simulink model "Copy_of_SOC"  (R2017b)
settings: Solver=FixedStepDiscrete  StartTime=0.0  StopTime=10.0  FixedStep=0.01  RelTol=1e-3  EnableMultiTasking=on
undefined symbols (not defined in the file): ASWTYPE_FALSE, ASWTYPE_TRUE, CaSOC_OneSOCVoltTable_mV, CaSOC_ZeroSOCTempTable_C, CaSOC_ZeroSOCVoltTable_mV, CbSOC_ManualDeplaCorrect_flg, CbSOC_ManuOCVCorrect_flg, CbSOC_SOCHighDiagOn_flg, CbSOC_SOCLowDiagOn_flg, CcSOC_ACChrgFinishDispSOC_pct, CcSOC_ACChrgFinishMaxSOC_pct, CcSOC_ACStepChrgMaxSOC_pct, CcSOC_AllowMaxCellSOC_pct, CcSOC_AllowMinCellSOC_pct, CcSOC_CapCalcCycl_ms, CcSOC_CellMinTempFilterAvg_numb, CcSOC_CellVoltMeasTol_mV, CcSOC_ChrgFishBefMaxSOC_pct, CcSOC_ChrgFishBefMinSOC_pct, CcSOC_ChrgFollowCurr_A, CcSOC_DCChrgFinishDispSOC_pct, CcSOC_DCChrgFinishMaxSOC_pct, CcSOC_DCStepChrgMaxSOC_pct, CcSOC_DeplaCellVoltMeasTol_mV, CcSOC_DeplaCorrectSOCDiff_pct, CcSOC_DisChrgFlwCurr_A, CcSOC_DispSOCChgSleepTime_min, CcSOC_DispSOCCordRunTi_ms, CcSOC_DispSOCErr_pct, CcSOC_FlwTarSOCDiff_pct, CcSOC_FullChrgTempThrld_C, CcSOC_MaxFlwDispSOC_pct, CcSOC_MinFlwDispSOC_pct, CcSOC_OCVCorrectRunTime_ms, CcSOC_OCVCorrectSleepTime_min, CcSOC_OCVCorrectSOCDiff_pct, CcSOC_OCVPeakCellVoltDev_mV, CcSOC_OCVPeakCellVoltTime_ms, CcSOC_PackSOCUseMax_pct, CcSOC_PackSOCUseMin_pct, CcSOC_SOCDeplaCurrThrd_A, CcSOC_SOCDeplaCurrThrdTi_ms, CcSOC_SOCDeplaNoOCVTi_min, CcSOC_SOCDeplaOCVTi_min, CcSOC_SOCHighAlarmThrld_pct, CcSOC_SOCHighWarningThrld_pct, CcSOC_SOCHysValue_pct, CcSOC_SOCLowAlarmThrld_pct, CcSOC_SOCLowWarningThrld_pct, CcSOC_ZeroMinSOC_pct, CcSOC_ZeroPackCrntThrd_A, CcSOC_ZeroSOCRunTime_ms, Enum_CTCCtrCtlConnMode, Enum_MSMBMUState, SOC_CONST0_NUMB, SOC_CONST1000_NUMB, SOC_CONST100_NUMB, SOC_CONST2080_NUMB, SOC_CONST3600000_NUMB, SOC_CONST60000_NUMB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
libraries: AIWAYS_Powertrain_BMS_lib x109
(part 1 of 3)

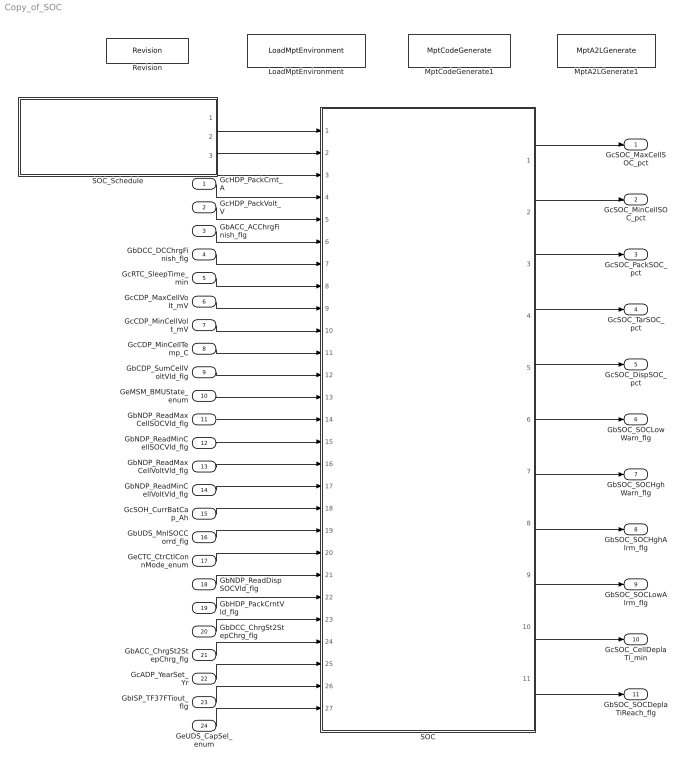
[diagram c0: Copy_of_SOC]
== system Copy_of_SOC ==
  GcHDP_PackCrnt_A : Inport
  GcHDP_PackVolt_V : Inport  Port=2
  GbACC_ACChrgFinish_flg : Inport  Port=3
  GbDCC_DCChrgFinish_flg : Inport  Port=4
  GcRTC_SleepTime_min : Inport  Port=5
  GcCDP_MaxCellVolt_mV : Inport  Port=6
  GcCDP_MinCellVolt_mV : Inport  Port=7
  GcCDP_MinCellTemp_C : Inport  Port=8
  GbCDP_SumCellVoltVld_flg : Inport  Port=9
  GeMSM_BMUState_enum : Inport  Port=10
  GbNDP_ReadMaxCellSOCVld_flg : Inport  Port=11
  GbNDP_ReadMinCellSOCVld_flg : Inport  Port=12
  GbNDP_ReadMaxCellVoltVld_flg : Inport  Port=13
  GbNDP_ReadMinCellVoltVld_flg : Inport  Port=14
  GcSOH_CurrBatCap_Ah : Inport  Port=15
  GbUDS_MnlSOCCorrd_flg : Inport  Port=16
  GeCTC_CtrCtlConnMode_enum : Inport  Port=17
  GbNDP_ReadDispSOCVld_flg : Inport  Port=18
  GbHDP_PackCrntVld_flg : Inport  Port=19
  GbDCC_ChrgSt2StepChrg_flg : Inport  Port=20
  GbACC_ChrgSt2StepChrg_flg : Inport  Port=21
  GcADP_YearSet_Yr : Inport  Port=22
  GbISP_TF37FTiout_flg : Inport  Port=23
  GeUDS_CapSel_enum : Inport  Port=24
  LoadMptEnvironment : AIWAYS_Powertrain_BMS_lib/Config/LoadMptEnvironment  ProjectName=Comm  SuppierID=NewPlatformUAES
  MptA2LGenerate1 : AIWAYS_Powertrain_BMS_lib/Config/MptA2LGenerate  SystemSampleTime=-1
  MptCodeGenerate1 : AIWAYS_Powertrain_BMS_lib/Config/MptCodeGenerate  SystemSampleTime=-1
  Revision : AIWAYS_Powertrain_BMS_lib/Config/Revision  curVersion='M110C113'  newVersion='M110C113'
  SOC : Subsystem
  SOC_Schedule : Stateflow chart  TreatAsAtomicUnit=on
  GcSOC_MaxCellSOC_pct : Outport
  GcSOC_MinCellSOC_pct : Outport  Port=2
  GcSOC_PackSOC_pct : Outport  Port=3
  GcSOC_TarSOC_pct : Outport  Port=4
  GcSOC_DispSOC_pct : Outport  Port=5
  GbSOC_SOCLowWarn_flg : Outport  Port=6
  GbSOC_SOCHghWarn_flg : Outport  Port=7
  GbSOC_SOCHghAlrm_flg : Outport  Port=8
  GbSOC_SOCLowAlrm_flg : Outport  Port=9
  GcSOC_CellDeplaTi_min : Outport  Port=10
  GbSOC_SOCDeplaTiReach_flg : Outport  Port=11
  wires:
  SOC/4(GcSOC_TarSOC_pct) -> GcSOC_TarSOC_pct/1
  SOC/3(GcSOC_PackSOC_pct) -> GcSOC_PackSOC_pct/1
  SOC/1(GcSOC_MaxCellSOC_pct) -> GcSOC_MaxCellSOC_pct/1
  SOC/2(GcSOC_MinCellSOC_pct) -> GcSOC_MinCellSOC_pct/1
  SOC_Schedule/3(SOC_SOCDisp_100ms()) -> SOC/3(SOC_SOCDisp_100ms)
  SOC_Schedule/2(SOC_SOCCal_100ms()) -> SOC/2(SOC_SOCCal_100ms)
  SOC_Schedule/1(SOC_SOCOCV_10ms()) -> SOC/1(SOC_SOCOCV_10ms)
  GcHDP_PackCrnt_A/1 -> SOC/4(GcHDP_PackCrnt_A)
  GcHDP_PackVolt_V/1 -> SOC/5(GcHDP_PackVolt_V)
  GbACC_ACChrgFinish_flg/1 -> SOC/6(GbACC_ACChrgFinish_flg)
  GbDCC_DCChrgFinish_flg/1 -> SOC/7(GbDCC_DCChrgFinish_flg)
  GcRTC_SleepTime_min/1 -> SOC/8(GcRTC_SleepTime_min)
  GcCDP_MaxCellVolt_mV/1 -> SOC/9(GcCDP_MaxCellVolt_mV)
  GcCDP_MinCellVolt_mV/1 -> SOC/10(GcCDP_MinCellVolt_mV)
  GcCDP_MinCellTemp_C/1 -> SOC/11(GcCDP_MinCellTemp_C)
  GbCDP_SumCellVoltVld_flg/1 -> SOC/12(GbCDP_SumCellVoltVld_flg)
  GeMSM_BMUState_enum/1 -> SOC/13(GeMSM_BMUState_enum)
  GbNDP_ReadMaxCellSOCVld_flg/1 -> SOC/14(GbNDP_ReadMaxCellSOCVld_flg)
  GbNDP_ReadMinCellSOCVld_flg/1 -> SOC/15(GbNDP_ReadMinCellSOCVld_flg)
  GbNDP_ReadMaxCellVoltVld_flg/1 -> SOC/16(GbNDP_ReadMaxCellVoltVld_flg)
  GbNDP_ReadMinCellVoltVld_flg/1 -> SOC/17(GbNDP_ReadMinCellVoltVld_flg)
  GcSOH_CurrBatCap_Ah/1 -> SOC/18(GcSOH_CurrBatCap_Ah)
  GbUDS_MnlSOCCorrd_flg/1 -> SOC/19(GbUDS_MnlSOCCorrd_flg)
  GeCTC_CtrCtlConnMode_enum/1 -> SOC/20(GeCTC_CtrCtlConnMode_enum)
  SOC/5(GcSOC_DispSOC_pct) -> GcSOC_DispSOC_pct/1
  SOC/6(GbSOC_SOCLowWarn_flg) -> GbSOC_SOCLowWarn_flg/1
  SOC/9(GbSOC_SOCLowAlrm_flg) -> GbSOC_SOCLowAlrm_flg/1
  SOC/8(GbSOC_SOCHghAlrm_flg) -> GbSOC_SOCHghAlrm_flg/1
  SOC/7(GbSOC_SOCHghWarn_flg) -> GbSOC_SOCHghWarn_flg/1
  GbNDP_ReadDispSOCVld_flg/1 -> SOC/21(GbNDP_ReadDispSOCVld_flg)
  GbHDP_PackCrntVld_flg/1 -> SOC/22(GbHDP_PackCrntVld_flg)
  SOC/10(GcSOC_CellDeplaTi_min) -> GcSOC_CellDeplaTi_min/1
  SOC/11(GbSOC_SOCDeplaTiReach_flg) -> GbSOC_SOCDeplaTiReach_flg/1
  GbDCC_ChrgSt2StepChrg_flg/1 -> SOC/23(GbDCC_ChrgSt2StepChrg_flg)
  GbACC_ChrgSt2StepChrg_flg/1 -> SOC/24(GbACC_ChrgSt2StepChrg_flg)
  GcADP_YearSet_Yr/1 -> SOC/25(GcADP_YearSet_Yr)
  GbISP_TF37FTiout_flg/1 -> SOC/26(GbISP_TF37FTiout_flg)
  GeUDS_CapSel_enum/1 -> SOC/27(GeUDS_CapSel_enum)

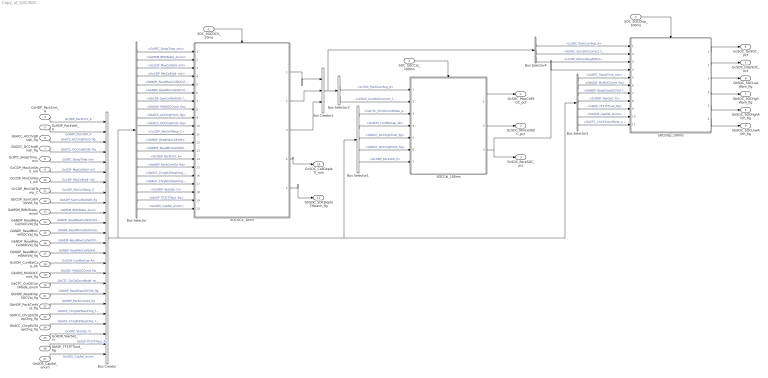
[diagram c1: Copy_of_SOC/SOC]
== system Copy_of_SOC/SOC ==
  SOC_SOCOCV_10ms : Inport
  SOC_SOCCal_100ms : Inport  Port=2
  SOC_SOCDisp_100ms : Inport  Port=3
  GcHDP_PackCrnt_A : Inport  Port=4
  GcHDP_PackVolt_V : Inport  Port=5
  GbACC_ACChrgFinish_flg : Inport  Port=6
  GbDCC_DCChrgFinish_flg : Inport  Port=7
  GcRTC_SleepTime_min : Inport  Port=8
  GcCDP_MaxCellVolt_mV : Inport  Port=9
  GcCDP_MinCellVolt_mV : Inport  Port=10
  GcCDP_MinCellTemp_C : Inport  Port=11
  GbCDP_SumCellVoltVld_flg : Inport  Port=12
  GeMSM_BMUState_enum : Inport  Port=13
  GbNDP_ReadMaxCellSOCVld_flg : Inport  Port=14
  GbNDP_ReadMinCellSOCVld_flg : Inport  Port=15
  GbNDP_ReadMaxCellVoltVld_flg : Inport  Port=16
  GbNDP_ReadMinCellVoltVld_flg : Inport  Port=17
  GcSOH_CurrBatCap_Ah : Inport  Port=18
  GbUDS_MnlSOCCorrd_flg : Inport  Port=19
  GeCTC_CtrCtlConnMode_enum : Inport  Port=20
  GbNDP_ReadDispSOCVld_flg : Inport  Port=21
  GbHDP_PackCrntVld_flg : Inport  Port=22
  GbDCC_ChrgSt2StepChrg_flg : Inport  Port=23
  GbACC_ChrgSt2StepChrg_flg : Inport  Port=24
  GcADP_YearSet_Yr : Inport  Port=25
  GbISP_TF37FTiout_flg : Inport  Port=26
  GeUDS_CapSel_enum : Inport  Port=27
  Bus Creator : BusCreator  Inputs=24
  Bus Creator1 : BusCreator  Inputs=3
  Bus Selector : BusSelector  OutputSignals=GcRTC_SleepTime_min,GeMSM_BMUState_enum,GcCDP_MaxCellVolt_mV,GcCDP_MinCellVolt_mV,GbNDP_ReadMaxCellSOCVld_flg,GbNDP_ReadMinCellSOCVld_flg,GbCDP_SumCellVoltVld_flg,GbUDS_MnlSOCCorrd_flg,GbACC_ACChrgFinish_flg,GbDCC_DCChrgFinish_flg,GcCDP_MinCellTemp_C,GbNDP_ReadMaxCellVoltVld_flg,GbNDP_ReadMinCellVoltVld_flg,GcHDP_PackCrnt_A,GbHDP_PackCrntVld_flg,GbDCC_ChrgSt2StepChrg_flg,GbACC_ChrgSt2StepChrg_flg,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
  Bus Selector1 : BusSelector  OutputSignals=GeCTC_CtrCtlConnMode_enum,GcSOH_CurrBatCap_Ah,GbACC_ACChrgFinish_flg,GbDCC_DCChrgFinish_flg,GcHDP_PackVolt_V
  Bus Selector2 : BusSelector  OutputSignals=GcRTC_SleepTime_min,GbUDS_MnlSOCCorrd_flg,GbNDP_ReadDispSOCVld_flg,GcADP_YearSet_Yr,GbISP_TF37FTiout_flg,GeUDS_CapSel_enum,GeCTC_CtrCtlConnMode_enum
  Bus Selector3 : BusSelector  OutputSignals=LcSOC_PackCurrAvg_A,LbSOC_ZeroSOCCorrect_flg
  Bus Selector4 : BusSelector  OutputSignals=LcSOC_PackCurrAvg_A,LbSOC_ZeroSOCCorrect_flg,LcCDP_MinCellAvgFitTemp_C
  SOCCal_100ms : Subsystem
  SOCDisp_100ms : Subsystem
  SOCOCV_10ms : Subsystem
  GcSOC_MaxCellSOC_pct : Outport
  GcSOC_MinCellSOC_pct : Outport  Port=2
  GcSOC_PackSOC_pct : Outport  Port=3
  GcSOC_TarSOC_pct : Outport  Port=4
  GcSOC_DispSOC_pct : Outport  Port=5
  GbSOC_SOCLowWarn_flg : Outport  Port=6
  GbSOC_SOCHghWarn_flg : Outport  Port=7
  GbSOC_SOCHghAlrm_flg : Outport  Port=8
  GbSOC_SOCLowAlrm_flg : Outport  Port=9
  GcSOC_CellDeplaTi_min : Outport  Port=10
  GbSOC_SOCDeplaTiReach_flg : Outport  Port=11
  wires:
  SOC_SOCDisp_100ms/1 -> SOCDisp_100ms/Trigger
  SOC_SOCCal_100ms/1 -> SOCCal_100ms/Trigger
  SOC_SOCOCV_10ms/1 -> SOCOCV_10ms/Trigger
  Bus Selector/1 -> SOCOCV_10ms/1(GcRTC_SleepTime_min)  "<GcRTC_SleepTime_min>"
  Bus Selector/2 -> SOCOCV_10ms/2(GeMSM_BMUState_enum)  "<GeMSM_BMUState_enum>"
  Bus Selector/3 -> SOCOCV_10ms/3(GcCDP_MaxCellVolt_mV)  "<GcCDP_MaxCellVolt_mV>"
  Bus Selector/4 -> SOCOCV_10ms/4(GcCDP_MinCellVolt_mV)  "<GcCDP_MinCellVolt_mV>"
  Bus Selector/5 -> SOCOCV_10ms/5(GbNDP_ReadMaxCellSOCVld_flg)  "<GbNDP_ReadMaxCellSOCVld_flg>"
  Bus Selector/6 -> SOCOCV_10ms/6(GbNDP_ReadMinCellSOCVld_flg)  "<GbNDP_ReadMinCellSOCVld_flg>"
  Bus Selector/7 -> SOCOCV_10ms/7(GbCDP_SumCellVoltVld_flg)  "<GbCDP_SumCellVoltVld_flg>"
  Bus Selector/8 -> SOCOCV_10ms/8(GbUDS_MnlSOCCorrd_flg)  "<GbUDS_MnlSOCCorrd_flg>"
  Bus Selector/9 -> SOCOCV_10ms/9(GbACC_ACChrgFinish_flg)  "<GbACC_ACChrgFinish_flg>"
  Bus Selector/10 -> SOCOCV_10ms/10(GbDCC_DCChrgFinish_flg)  "<GbDCC_DCChrgFinish_flg>"
  Bus Selector/11 -> SOCOCV_10ms/11(GcCDP_MinCellTemp_C)  "<GcCDP_MinCellTemp_C>"
  Bus Selector/12 -> SOCOCV_10ms/12(GbNDP_ReadMaxCellVoltVld_flg)  "<GbNDP_ReadMaxCellVoltVld_flg>"
  Bus Selector/13 -> SOCOCV_10ms/13(GbNDP_ReadMinCellVoltVld_flg)  "<GbNDP_ReadMinCellVoltVld_flg>"
  Bus Selector/14 -> SOCOCV_10ms/14(GcHDP_PackCrnt_A)  "<GcHDP_PackCrnt_A>"
  GcHDP_PackCrnt_A/1 -> Bus Creator/1  "GcHDP_PackCrnt_A"
  GcHDP_PackVolt_V/1 -> Bus Creator/2  "GcHDP_PackVolt_V"
  GbACC_ACChrgFinish_flg/1 -> Bus Creator/3  "GbACC_ACChrgFinish_flg"
  GbDCC_DCChrgFinish_flg/1 -> Bus Creator/4  "GbDCC_DCChrgFinish_flg"
  GcRTC_SleepTime_min/1 -> Bus Creator/5  "GcRTC_SleepTime_min"
  GcCDP_MaxCellVolt_mV/1 -> Bus Creator/6  "GcCDP_MaxCellVolt_mV"
  GcCDP_MinCellVolt_mV/1 -> Bus Creator/7  "GcCDP_MinCellVolt_mV"
  GcCDP_MinCellTemp_C/1 -> Bus Creator/8  "GcCDP_MinCellTemp_C"
  GbCDP_SumCellVoltVld_flg/1 -> Bus Creator/9  "GbCDP_SumCellVoltVld_flg"
  GeMSM_BMUState_enum/1 -> Bus Creator/10  "GeMSM_BMUState_enum"
  GbNDP_ReadMaxCellSOCVld_flg/1 -> Bus Creator/11  "GbNDP_ReadMaxCellSOCVld_flg"
  GbNDP_ReadMinCellSOCVld_flg/1 -> Bus Creator/12  "GbNDP_ReadMinCellSOCVld_flg"
  GbNDP_ReadMaxCellVoltVld_flg/1 -> Bus Creator/13  "GbNDP_ReadMaxCellVoltVld_flg"
  GbNDP_ReadMinCellVoltVld_flg/1 -> Bus Creator/14  "GbNDP_ReadMinCellVoltVld_flg"
  GcSOH_CurrBatCap_Ah/1 -> Bus Creator/15  "GcSOH_CurrBatCap_Ah"
  GbUDS_MnlSOCCorrd_flg/1 -> Bus Creator/16  "GbUDS_MnlSOCCorrd_flg"
  GeCTC_CtrCtlConnMode_enum/1 -> Bus Creator/17  "GeCTC_CtrCtlConnMode_enum"
  Bus Creator/1 -> Bus Selector2/1, Bus Selector1/1, Bus Selector/1
  Bus Selector1/1 -> SOCCal_100ms/3(GeCTC_CtrCtlConnMode_enum)  "<GeCTC_CtrCtlConnMode_enum>"
  Bus Selector1/2 -> SOCCal_100ms/4(GcSOH_CurrBatCap_Ah)  "<GcSOH_CurrBatCap_Ah>"
  Bus Selector1/3 -> SOCCal_100ms/5(GbACC_ACChrgFinish_flg)  "<GbACC_ACChrgFinish_flg>"
  Bus Selector1/4 -> SOCCal_100ms/6(GbDCC_DCChrgFinish_flg)  "<GbDCC_DCChrgFinish_flg>"
  Bus Selector1/5 -> SOCCal_100ms/7(GcHDP_PackVolt_V)  "<GcHDP_PackVolt_V>"
  SOCCal_100ms/3(GcSOC_PackSOC_pct) -> SOCDisp_100ms/4(GcSOC_PackSOC_pct), GcSOC_PackSOC_pct/1
  Bus Selector2/1 -> SOCDisp_100ms/5(GcRTC_SleepTime_min)  "<GcRTC_SleepTime_min>"
  Bus Selector2/2 -> SOCDisp_100ms/6(GbUDS_MnlSOCCorrd_flg)  "<GbUDS_MnlSOCCorrd_flg>"
  SOCCal_100ms/1(GcSOC_MaxCellSOC_pct) -> GcSOC_MaxCellSOC_pct/1
  SOCCal_100ms/2(GcSOC_MinCellSOC_pct) -> GcSOC_MinCellSOC_pct/1
  SOCDisp_100ms/1(GcSOC_TarSOC_pct) -> GcSOC_TarSOC_pct/1
  SOCDisp_100ms/2(GcSOC_DispSOC_pct) -> GcSOC_DispSOC_pct/1
  SOCDisp_100ms/3(GbSOC_SOCLowWarn_flg) -> GbSOC_SOCLowWarn_flg/1
  SOCDisp_100ms/4(GbSOC_SOCHghWarn_flg) -> GbSOC_SOCHghWarn_flg/1
  SOCDisp_100ms/5(GbSOC_SOCHghAlrm_flg) -> GbSOC_SOCHghAlrm_flg/1
  SOCDisp_100ms/6(GbSOC_SOCLowAlrm_flg) -> GbSOC_SOCLowAlrm_flg/1
  GbNDP_ReadDispSOCVld_flg/1 -> Bus Creator/18  "GbNDP_ReadDispSOCVld_flg"
  Bus Selector2/3 -> SOCDisp_100ms/7(GbNDP_ReadDispSOCVld_flg)  "<GbNDP_ReadDispSOCVld_flg>"
  GbHDP_PackCrntVld_flg/1 -> Bus Creator/19  "GbHDP_PackCrntVld_flg"
  Bus Selector/15 -> SOCOCV_10ms/15(GbHDP_PackCrntVld_flg)  "<GbHDP_PackCrntVld_flg>"
  SOCOCV_10ms/4(GcSOC_CellDeplaTi_min) -> GcSOC_CellDeplaTi_min/1
  SOCOCV_10ms/5(GbSOC_SOCDeplaTiReach_flg) -> GbSOC_SOCDeplaTiReach_flg/1
  SOCOCV_10ms/1(LcSOC_PackCurrAvg_A) -> Bus Creator1/1
  SOCOCV_10ms/2(LbSOC_ZeroSOCCorrect_flg) -> Bus Creator1/2
  Bus Creator1/1 -> Bus Selector4/1, Bus Selector3/1
  Bus Selector3/1 -> SOCCal_100ms/1(LcSOC_PackCurrAvg_A)  "<LcSOC_PackCurrAvg_A>"
  Bus Selector3/2 -> SOCCal_100ms/2(LbSOC_ZeroSOCCorrect_flg)  "<LbSOC_ZeroSOCCorrect_flg>"
  Bus Selector4/1 -> SOCDisp_100ms/1(LcSOC_PackCurrAvg_A)  "<LcSOC_PackCurrAvg_A>"
  Bus Selector4/2 -> SOCDisp_100ms/2(LbSOC_ZeroSOCCorrect_flg)  "<LbSOC_ZeroSOCCorrect_flg>"
  GbDCC_ChrgSt2StepChrg_flg/1 -> Bus Creator/20  "GbDCC_ChrgSt2StepChrg_flg"
  GbACC_ChrgSt2StepChrg_flg/1 -> Bus Creator/21  "GbACC_ChrgSt2StepChrg_flg"
  Bus Selector/16 -> SOCOCV_10ms/16(GbDCC_ChrgSt2StepChrg_flg)  "<GbDCC_ChrgSt2StepChrg_flg>"
  Bus Selector/17 -> SOCOCV_10ms/17(GbACC_ChrgSt2StepChrg_flg)  "<GbACC_ChrgSt2StepChrg_flg>"
  SOCOCV_10ms/3(LcCDP_MinCellAvgFitTemp_C) -> Bus Creator1/3
  Bus Selector4/3 -> SOCDisp_100ms/3(LcCDP_MinCellAvgFitTemp_C)  "<LcCDP_MinCellAvgFitTemp_C>"
  GcADP_YearSet_Yr/1 -> Bus Creator/22  "GcADP_YearSet_Yr"
  GbISP_TF37FTiout_flg/1 -> Bus Creator/23  "GbISP_TF37FTiout_flg"
  Bus Selector/18 -> SOCOCV_10ms/18(GcADP_YearSet_Yr)  "<GcADP_YearSet_Yr>"
  Bus Selector/19 -> SOCOCV_10ms/19(GbISP_TF37FTiout_flg)  "<GbISP_TF37FTiout_flg>"
  Bus Selector2/4 -> SOCDisp_100ms/8(GcADP_YearSet_Yr)  "<GcADP_YearSet_Yr>"
  Bus Selector2/5 -> SOCDisp_100ms/9(GbISP_TF37FTiout_flg)  "<GbISP_TF37FTiout_flg>"
  GeUDS_CapSel_enum/1 -> Bus Creator/24  "GeUDS_CapSel_enum"
  Bus Selector/20 -> SOCOCV_10ms/20(GeUDS_CapSel_enum)  "<GeUDS_CapSel_enum>"
  Bus Selector2/6 -> SOCDisp_100ms/10(GeUDS_CapSel_enum)  "<GeUDS_CapSel_enum>"
  Bus Selector2/7 -> SOCDisp_100ms/11(GeCTC_CtrCtlConnMode_enum)  "<GeCTC_CtrCtlConnMode_enum>"

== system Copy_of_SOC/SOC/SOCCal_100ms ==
  LcSOC_PackCurrAvg_A : Inport
  LbSOC_ZeroSOCCorrect_flg : Inport  Port=2
  GeCTC_CtrCtlConnMode_enum : Inport  Port=3
  GcSOH_CurrBatCap_Ah : Inport  Port=4
  GbACC_ACChrgFinish_flg : Inport  Port=5
  GbDCC_DCChrgFinish_flg : Inport  Port=6
  GcHDP_PackVolt_V : Inport  Port=7
  SOC_SOCCal_100ms : TriggerPort  TriggerType=function-call  VariantControl=(inherit)
  SOCCal_100ms_sys : Subsystem
  GcSOC_MaxCellSOC_pct : Outport
  GcSOC_MinCellSOC_pct : Outport  Port=2
  GcSOC_PackSOC_pct : Outport  Port=3
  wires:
  LcSOC_PackCurrAvg_A/1 -> SOCCal_100ms_sys/1(LcSOC_PackCurrAvg_A)
  GeCTC_CtrCtlConnMode_enum/1 -> SOCCal_100ms_sys/3(GeCTC_CtrCtlConnMode_enum)
  GcSOH_CurrBatCap_Ah/1 -> SOCCal_100ms_sys/4(GcSOH_CurrBatCap_Ah)
  GbACC_ACChrgFinish_flg/1 -> SOCCal_100ms_sys/5(GbACC_ACChrgFinish_flg)
  GbDCC_DCChrgFinish_flg/1 -> SOCCal_100ms_sys/6(GbDCC_DCChrgFinish_flg)
  GcHDP_PackVolt_V/1 -> SOCCal_100ms_sys/7(GcHDP_PackVolt_V)
  SOCCal_100ms_sys/1(GcSOC_MaxCellSOC_pct) -> GcSOC_MaxCellSOC_pct/1
  SOCCal_100ms_sys/2(GcSOC_MinCellSOC_pct) -> GcSOC_MinCellSOC_pct/1
  SOCCal_100ms_sys/3(GcSOC_PackSOC_pct) -> GcSOC_PackSOC_pct/1
  LbSOC_ZeroSOCCorrect_flg/1 -> SOCCal_100ms_sys/2(LbSOC_ZeroSOCCorrect_flg)

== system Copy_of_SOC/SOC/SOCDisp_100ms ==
  LcSOC_PackCurrAvg_A : Inport
  LbSOC_ZeroSOCCorrect_flg : Inport  Port=2
  LcCDP_MinCellAvgFitTemp_C : Inport  Port=3
  GcSOC_PackSOC_pct : Inport  Port=4
  GcRTC_SleepTime_min : Inport  Port=5
  GbUDS_MnlSOCCorrd_flg : Inport  Port=6
  GbNDP_ReadDispSOCVld_flg : Inport  Port=7
  GcADP_YearSet_Yr : Inport  Port=8
  GbISP_TF37FTiout_flg : Inport  Port=9
  GeUDS_CapSel_enum : Inport  Port=10
  GeCTC_CtrCtlConnMode_enum : Inport  Port=11
  SOC_SOCDisp_100ms : TriggerPort  TriggerType=function-call  VariantControl=(inherit)
  SOCDisp_100ms_sys : Subsystem
  GcSOC_TarSOC_pct : Outport
  GcSOC_DispSOC_pct : Outport  Port=2
  GbSOC_SOCLowWarn_flg : Outport  Port=3
  GbSOC_SOCHghWarn_flg : Outport  Port=4
  GbSOC_SOCHghAlrm_flg : Outport  Port=5
  GbSOC_SOCLowAlrm_flg : Outport  Port=6
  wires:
  GcSOC_PackSOC_pct/1 -> SOCDisp_100ms_sys/4(GcSOC_PackSOC_pct)
  LcSOC_PackCurrAvg_A/1 -> SOCDisp_100ms_sys/1(LcSOC_PackCurrAvg_A)
  GcRTC_SleepTime_min/1 -> SOCDisp_100ms_sys/5(GcRTC_SleepTime_min)
  GbUDS_MnlSOCCorrd_flg/1 -> SOCDisp_100ms_sys/6(GbUDS_MnlSOCCorrd_flg)
  SOCDisp_100ms_sys/1(GcSOC_TarSOC_pct) -> GcSOC_TarSOC_pct/1
  SOCDisp_100ms_sys/2(GcSOC_DispSOC_pct) -> GcSOC_DispSOC_pct/1
  SOCDisp_100ms_sys/3(GbSOC_SOCLowWarn_flg) -> GbSOC_SOCLowWarn_flg/1
  SOCDisp_100ms_sys/4(GbSOC_SOCHghWarn_flg) -> GbSOC_SOCHghWarn_flg/1
  SOCDisp_100ms_sys/5(GbSOC_SOCHghAlrm_flg) -> GbSOC_SOCHghAlrm_flg/1
  SOCDisp_100ms_sys/6(GbSOC_SOCLowAlrm_flg) -> GbSOC_SOCLowAlrm_flg/1
  GbNDP_ReadDispSOCVld_flg/1 -> SOCDisp_100ms_sys/7(GbNDP_ReadDispSOCVld_flg)
  LbSOC_ZeroSOCCorrect_flg/1 -> SOCDisp_100ms_sys/2(LbSOC_ZeroSOCCorrect_flg)
  LcCDP_MinCellAvgFitTemp_C/1 -> SOCDisp_100ms_sys/3(LcCDP_MinCellAvgFitTemp_C)
  GcADP_YearSet_Yr/1 -> SOCDisp_100ms_sys/8(GcADP_YearSet_Yr)
  GbISP_TF37FTiout_flg/1 -> SOCDisp_100ms_sys/9(GbISP_TF37FTiout_flg)
  GeUDS_CapSel_enum/1 -> SOCDisp_100ms_sys/10(GeUDS_CapSel_enum)
  GeCTC_CtrCtlConnMode_enum/1 -> SOCDisp_100ms_sys/11(GeCTC_CtrCtlConnMode_enum)

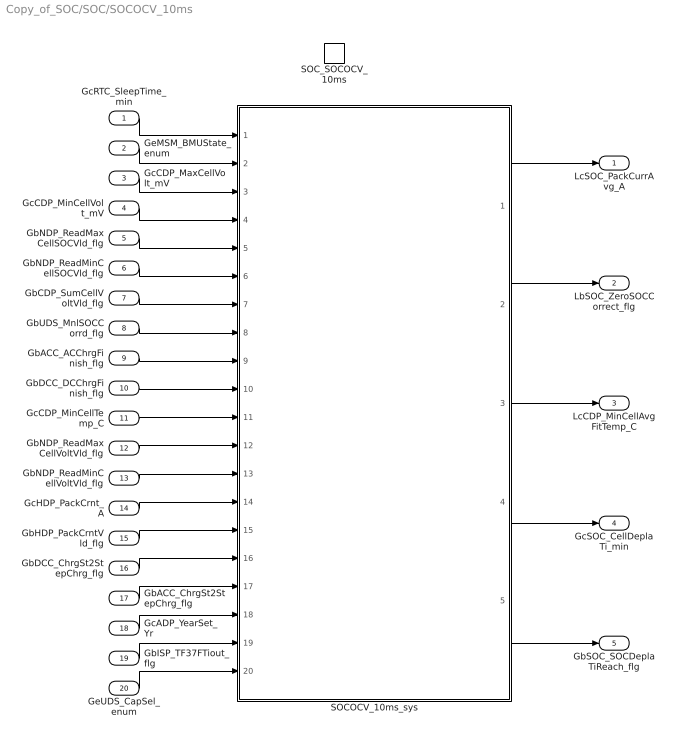
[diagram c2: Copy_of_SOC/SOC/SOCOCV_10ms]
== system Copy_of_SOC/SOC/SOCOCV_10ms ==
  GcRTC_SleepTime_min : Inport
  GeMSM_BMUState_enum : Inport  Port=2
  GcCDP_MaxCellVolt_mV : Inport  Port=3
  GcCDP_MinCellVolt_mV : Inport  Port=4
  GbNDP_ReadMaxCellSOCVld_flg : Inport  Port=5
  GbNDP_ReadMinCellSOCVld_flg : Inport  Port=6
  GbCDP_SumCellVoltVld_flg : Inport  Port=7
  GbUDS_MnlSOCCorrd_flg : Inport  Port=8
  GbACC_ACChrgFinish_flg : Inport  Port=9
  GbDCC_DCChrgFinish_flg : Inport  Port=10
  GcCDP_MinCellTemp_C : Inport  Port=11
  GbNDP_ReadMaxCellVoltVld_flg : Inport  Port=12
  GbNDP_ReadMinCellVoltVld_flg : Inport  Port=13
  GcHDP_PackCrnt_A : Inport  Port=14
  GbHDP_PackCrntVld_flg : Inport  Port=15
  GbDCC_ChrgSt2StepChrg_flg : Inport  Port=16
  GbACC_ChrgSt2StepChrg_flg : Inport  Port=17
  GcADP_YearSet_Yr : Inport  Port=18
  GbISP_TF37FTiout_flg : Inport  Port=19
  GeUDS_CapSel_enum : Inport  Port=20
  SOC_SOCOCV_10ms : TriggerPort  TriggerType=function-call  VariantControl=(inherit)
  SOCOCV_10ms_sys : Subsystem
  LcSOC_PackCurrAvg_A : Outport
  LbSOC_ZeroSOCCorrect_flg : Outport  Port=2
  LcCDP_MinCellAvgFitTemp_C : Outport  Port=3
  GcSOC_CellDeplaTi_min : Outport  Port=4
  GbSOC_SOCDeplaTiReach_flg : Outport  Port=5
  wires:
  GcRTC_SleepTime_min/1 -> SOCOCV_10ms_sys/1(GcRTC_SleepTime_min)
  GeMSM_BMUState_enum/1 -> SOCOCV_10ms_sys/2(GeMSM_BMUState_enum)
  GcCDP_MaxCellVolt_mV/1 -> SOCOCV_10ms_sys/3(GcCDP_MaxCellVolt_mV)
  GcCDP_MinCellVolt_mV/1 -> SOCOCV_10ms_sys/4(GcCDP_MinCellVolt_mV)
  GbNDP_ReadMaxCellSOCVld_flg/1 -> SOCOCV_10ms_sys/5(GbNDP_ReadMaxCellSOCVld_flg)
  GbNDP_ReadMinCellSOCVld_flg/1 -> SOCOCV_10ms_sys/6(GbNDP_ReadMinCellSOCVld_flg)
  GbCDP_SumCellVoltVld_flg/1 -> SOCOCV_10ms_sys/7(GbCDP_SumCellVoltVld_flg)
  GbUDS_MnlSOCCorrd_flg/1 -> SOCOCV_10ms_sys/8(GbUDS_MnlSOCCorrd_flg)
  GbACC_ACChrgFinish_flg/1 -> SOCOCV_10ms_sys/9(GbACC_ACChrgFinish_flg)
  GbDCC_DCChrgFinish_flg/1 -> SOCOCV_10ms_sys/10(GbDCC_DCChrgFinish_flg)
  GcCDP_MinCellTemp_C/1 -> SOCOCV_10ms_sys/11(GcCDP_MinCellTemp_C)
  GbNDP_ReadMaxCellVoltVld_flg/1 -> SOCOCV_10ms_sys/12(GbNDP_ReadMaxCellVoltVld_flg)
  GbNDP_ReadMinCellVoltVld_flg/1 -> SOCOCV_10ms_sys/13(GbNDP_ReadMinCellVoltVld_flg)
  GcHDP_PackCrnt_A/1 -> SOCOCV_10ms_sys/14(GcHDP_PackCrnt_A)
  SOCOCV_10ms_sys/1(LcSOC_PackCurrAvg_A) -> LcSOC_PackCurrAvg_A/1
  GbHDP_PackCrntVld_flg/1 -> SOCOCV_10ms_sys/15(GbHDP_PackCrntVld_flg)
  SOCOCV_10ms_sys/4(GcSOC_CellDeplaTi_min) -> GcSOC_CellDeplaTi_min/1
  SOCOCV_10ms_sys/5(GbSOC_SOCDeplaTiReach_flg) -> GbSOC_SOCDeplaTiReach_flg/1
  SOCOCV_10ms_sys/2(LbSOC_ZeroSOCCorrect_flg) -> LbSOC_ZeroSOCCorrect_flg/1
  GbDCC_ChrgSt2StepChrg_flg/1 -> SOCOCV_10ms_sys/16(GbDCC_ChrgSt2StepChrg_flg)
  GbACC_ChrgSt2StepChrg_flg/1 -> SOCOCV_10ms_sys/17(GbACC_ChrgSt2StepChrg_flg)
  SOCOCV_10ms_sys/3(LcCDP_MinCellAvgFitTemp_C) -> LcCDP_MinCellAvgFitTemp_C/1
  GcADP_YearSet_Yr/1 -> SOCOCV_10ms_sys/18(GcADP_YearSet_Yr)
  GbISP_TF37FTiout_flg/1 -> SOCOCV_10ms_sys/19(GbISP_TF37FTiout_flg)
  GeUDS_CapSel_enum/1 -> SOCOCV_10ms_sys/20(GeUDS_CapSel_enum)

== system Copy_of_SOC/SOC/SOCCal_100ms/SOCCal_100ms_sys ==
  LcSOC_PackCurrAvg_A : Inport
  LbSOC_ZeroSOCCorrect_flg : Inport  Port=2
  GeCTC_CtrCtlConnMode_enum : Inport  Port=3
  GcSOH_CurrBatCap_Ah : Inport  Port=4
  GbACC_ACChrgFinish_flg : Inport  Port=5
  GbDCC_DCChrgFinish_flg : Inport  Port=6
  GcHDP_PackVolt_V : Inport  Port=7
  CapPowerSum : Subsystem
  SOCCalculate : Subsystem
  GcSOC_MaxCellSOC_pct : Outport
  GcSOC_MinCellSOC_pct : Outport  Port=2
  GcSOC_PackSOC_pct : Outport  Port=3
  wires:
  GcHDP_PackVolt_V/1 -> CapPowerSum/1(GcHDP_PackVolt_V)
  SOCCalculate/3(GcSOC_PackSOC_pct) -> GcSOC_PackSOC_pct/1
  GcSOH_CurrBatCap_Ah/1 -> SOCCalculate/4(GcSOH_CurrBatCap_Ah)
  GbDCC_DCChrgFinish_flg/1 -> SOCCalculate/6(GbDCC_DCChrgFinish_flg)
  SOCCalculate/2(GcSOC_MinCellSOC_pct) -> GcSOC_MinCellSOC_pct/1
  GeCTC_CtrCtlConnMode_enum/1 -> SOCCalculate/3(GeCTC_CtrCtlConnMode_enum)
  GbACC_ACChrgFinish_flg/1 -> SOCCalculate/5(GbACC_ACChrgFinish_flg)
  SOCCalculate/1(GcSOC_MaxCellSOC_pct) -> GcSOC_MaxCellSOC_pct/1
  LcSOC_PackCurrAvg_A/1 -> SOCCalculate/1(LcSOC_PackCurrAvg_A), CapPowerSum/2(LcSOC_PackCurrAvg_A)
  LbSOC_ZeroSOCCorrect_flg/1 -> SOCCalculate/2(LbSOC_ZeroSOCCorrect_flg)

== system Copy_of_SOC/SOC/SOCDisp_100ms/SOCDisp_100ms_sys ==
  LcSOC_PackCurrAvg_A : Inport
  LbSOC_ZeroSOCCorrect_flg : Inport  Port=2
  LcCDP_MinCellAvgFitTemp_C : Inport  Port=3
  GcSOC_PackSOC_pct : Inport  Port=4
  GcRTC_SleepTime_min : Inport  Port=5
  GbUDS_MnlSOCCorrd_flg : Inport  Port=6
  GbNDP_ReadDispSOCVld_flg : Inport  Port=7
  GcADP_YearSet_Yr : Inport  Port=8
  GbISP_TF37FTiout_flg : Inport  Port=9
  GeUDS_CapSel_enum : Inport  Port=10
  GeCTC_CtrCtlConnMode_enum : Inport  Port=11
  SOCDisplay : Subsystem
  SOCWarningFlt : Subsystem
  GcSOC_TarSOC_pct : Outport
  GcSOC_DispSOC_pct : Outport  Port=2
  GbSOC_SOCLowWarn_flg : Outport  Port=3
  GbSOC_SOCHghWarn_flg : Outport  Port=4
  GbSOC_SOCHghAlrm_flg : Outport  Port=5
  GbSOC_SOCLowAlrm_flg : Outport  Port=6
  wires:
  SOCDisplay/2(GcSOC_DispSOC_pct) -> GcSOC_DispSOC_pct/1, SOCWarningFlt/1(GcSOC_DispSOC_pct)
  SOCDisplay/1(GcSOC_TarSOC_pct) -> GcSOC_TarSOC_pct/1
  GcSOC_PackSOC_pct/1 -> SOCDisplay/4(GcSOC_PackSOC_pct)
  LcSOC_PackCurrAvg_A/1 -> SOCDisplay/1(LcSOC_PackCurrAvg_A)
  GbUDS_MnlSOCCorrd_flg/1 -> SOCDisplay/6(GbUDS_MnlSOCCorrd_flg)
  GcRTC_SleepTime_min/1 -> SOCDisplay/5(GcRTC_SleepTime_min)
  GbNDP_ReadDispSOCVld_flg/1 -> SOCDisplay/7(GbNDP_ReadDispSOCVld_flg)
  LbSOC_ZeroSOCCorrect_flg/1 -> SOCDisplay/2(LbSOC_ZeroSOCCorrect_flg)
  LcCDP_MinCellAvgFitTemp_C/1 -> SOCDisplay/3(LcCDP_MinCellAvgFitTemp_C)
  GcADP_YearSet_Yr/1 -> SOCDisplay/8(GcADP_YearSet_Yr)
  GbISP_TF37FTiout_flg/1 -> SOCDisplay/9(GbISP_TF37FTiout_flg)
  SOCWarningFlt/1(GbSOC_SOCLowWarn_flg) -> GbSOC_SOCLowWarn_flg/1
  SOCWarningFlt/2(GbSOC_SOCHghWarn_flg) -> GbSOC_SOCHghWarn_flg/1
  SOCWarningFlt/3(GbSOC_SOCHghAlrm_flg) -> GbSOC_SOCHghAlrm_flg/1
  SOCWarningFlt/4(GbSOC_SOCLowAlrm_flg) -> GbSOC_SOCLowAlrm_flg/1
  GeUDS_CapSel_enum/1 -> SOCDisplay/10(GeUDS_CapSel_enum)
  GeCTC_CtrCtlConnMode_enum/1 -> SOCDisplay/11(GeCTC_CtrCtlConnMode_enum)

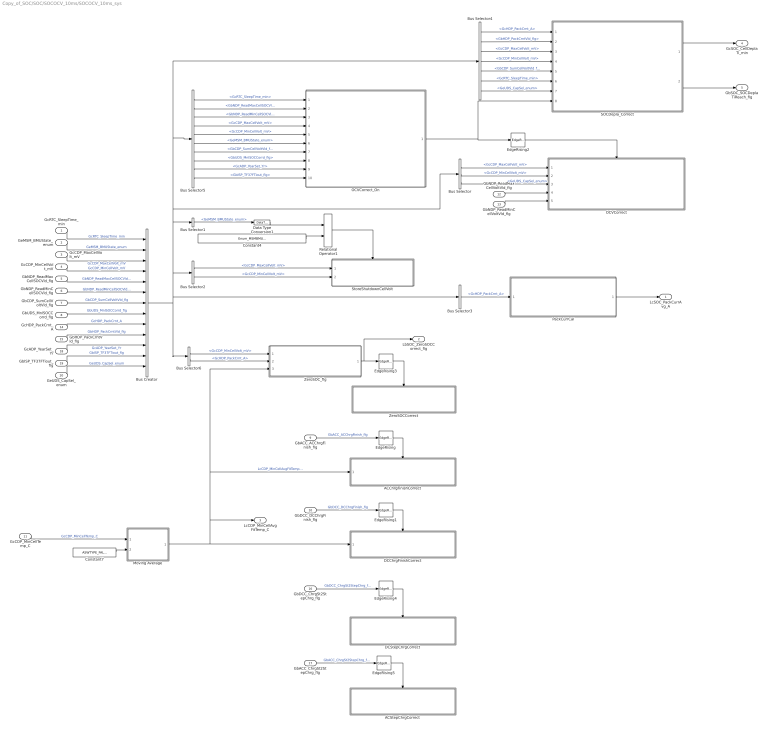
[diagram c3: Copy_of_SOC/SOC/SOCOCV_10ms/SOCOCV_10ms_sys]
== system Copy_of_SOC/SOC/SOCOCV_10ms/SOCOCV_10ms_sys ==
  GcRTC_SleepTime_min : Inport
  GeMSM_BMUState_enum : Inport  Port=2
  GcCDP_MaxCellVolt_mV : Inport  Port=3
  GcCDP_MinCellVolt_mV : Inport  Port=4
  GbNDP_ReadMaxCellSOCVld_flg : Inport  Port=5
  GbNDP_ReadMinCellSOCVld_flg : Inport  Port=6
  GbCDP_SumCellVoltVld_flg : Inport  Port=7
  GbUDS_MnlSOCCorrd_flg : Inport  Port=8
  GbACC_ACChrgFinish_flg : Inport  Port=9
  GbDCC_DCChrgFinish_flg : Inport  Port=10
  GcCDP_MinCellTemp_C : Inport  Port=11
  GbNDP_ReadMaxCellVoltVld_flg : Inport  Port=12
  GbNDP_ReadMinCellVoltVld_flg : Inport  Port=13
  GcHDP_PackCrnt_A : Inport  Port=14
  GbHDP_PackCrntVld_flg : Inport  Port=15
  GbDCC_ChrgSt2StepChrg_flg : Inport  Port=16
  GbACC_ChrgSt2StepChrg_flg : Inport  Port=17
  GcADP_YearSet_Yr : Inport  Port=18
  GbISP_TF37FTiout_flg : Inport  Port=19
  GeUDS_CapSel_enum : Inport  Port=20
  ACChrgFinishCorrect : Subsystem
  ACStepChrgCorrect : Subsystem
  Bus Creator : BusCreator  Inputs=13
  Bus Selector : BusSelector  OutputSignals=GcCDP_MaxCellVolt_mV,GcCDP_MinCellVolt_mV,GeUDS_CapSel_enum
  Bus Selector1 : BusSelector  OutputSignals=GeMSM_BMUState_enum
  Bus Selector2 : BusSelector  OutputSignals=GcCDP_MaxCellVolt_mV,GcCDP_MinCellVolt_mV
  Bus Selector3 : BusSelector  OutputSignals=GcHDP_PackCrnt_A
  Bus Selector4 : BusSelector  OutputSignals=GcHDP_PackCrnt_A,GbHDP_PackCrntVld_flg,GcCDP_MaxCellVolt_mV,GcCDP_MinCellVolt_mV,GbCDP_SumCellVoltVld_flg,GcRTC_SleepTime_min,GeUDS_CapSel_enum
  Bus Selector5 : BusSelector  OutputSignals=GcRTC_SleepTime_min,GbNDP_ReadMaxCellSOCVld_flg,GbNDP_ReadMinCellSOCVld_flg,GcCDP_MaxCellVolt_mV,GcCDP_MinCellVolt_mV,GeMSM_BMUState_enum,GbCDP_SumCellVoltVld_flg,GbUDS_MnlSOCCorrd_flg,GcADP_YearSet_Yr,GbISP_TF37FTiout_flg
  Bus Selector6 : BusSelector  OutputSignals=GcCDP_MinCellVolt_mV,GcHDP_PackCrnt_A
  Constant4 : Constant  Value=Enum_MSMBMUState.Enum_MSMBMUState_Shutdown
  Constant7 : Constant  Value=ASWTYPE_FALSE
  DCChrgFinishCorrect : Subsystem
  DCStepChrgCorrect : Subsystem
  Data Type Conversion1 : DataTypeConversion
  EdgeRising{,1..5} (6 alike) : AIWAYS_Powertrain_BMS_lib/Logical Operators/EdgeRising
  Moving Average : Subsystem  TreatAsAtomicUnit=on  mask(MovingAverage00){BufferSize=CcSOC_CellMinTempFilterAvg_numb}
      mask prompts: BufferSize "Buffer size"
      mask help: Block will compute the moving average of the input signal based on the number of samples input as the buffer_size. NOTE: Will not work with vectorized inputs. Default buffer size = 2. Input1=Value; Input2=Reset
  OCVCorrect : Subsystem
  OCVCorrect_On : Subsystem
  PackCurrCal : Subsystem
  Relational Operator1 : RelationalOperator  Operator===  OutDataTypeStr=boolean
  SOCDepla_Correct : Subsystem  TreatAsAtomicUnit=on
  StoreShutdownCellVolt : Subsystem  TreatAsAtomicUnit=on
  ZeroSOCCorrect : Subsystem
  ZeroSOC_flg : Subsystem
  LcSOC_PackCurrAvg_A : Outport
  LbSOC_ZeroSOCCorrect_flg : Outport  Port=2
  LcCDP_MinCellAvgFitTemp_C : Outport  Port=3
  GcSOC_CellDeplaTi_min : Outport  Port=4
  GbSOC_SOCDeplaTiReach_flg : Outport  Port=5
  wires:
  Data Type Conversion1/1 -> Relational Operator1/1
  GbNDP_ReadMaxCellVoltVld_flg/1 -> OCVCorrect/4(GbNDP_ReadMaxCellVoltVld_flg)
  Constant4/1 -> Relational Operator1/2
  GbDCC_DCChrgFinish_flg/1 -> EdgeRising1/1  "GbDCC_DCChrgFinish_flg"
  Bus Selector2/1 -> StoreShutdownCellVolt/1(GcCDP_MaxCellVolt_mV)  "<GcCDP_MaxCellVolt_mV>"
  Bus Selector1/1 -> Data Type Conversion1/1  "<GeMSM_BMUState_enum>"
  Bus Creator/1 -> Bus Selector2/1, Bus Selector1/1, Bus Selector4/1, Bus Selector5/1, Bus Selector/1, Bus Selector3/1, Bus Selector6/1
  GbACC_ACChrgFinish_flg/1 -> EdgeRising/1  "GbACC_ACChrgFinish_flg"
  Bus Selector/1 -> OCVCorrect/1(GcCDP_MaxCellVolt_mV)  "<GcCDP_MaxCellVolt_mV>"
  EdgeRising1/1 -> DCChrgFinishCorrect/Enable
  EdgeRising2/1 -> OCVCorrect/Enable
  EdgeRising/1 -> ACChrgFinishCorrect/Enable
  Bus Selector/2 -> OCVCorrect/2(GcCDP_MinCellVolt_mV)  "<GcCDP_MinCellVolt_mV>"
  Bus Selector2/2 -> StoreShutdownCellVolt/2(GcCDP_MinCellVolt_mV)  "<GcCDP_MinCellVolt_mV>"
  Relational Operator1/1 -> StoreShutdownCellVolt/Enable
  OCVCorrect_On/1(LbSOC_OCVCorrectOn_flg) -> SOCDepla_Correct/8(LbSOC_OCVCorrectOn_flg), EdgeRising2/1
  GbNDP_ReadMinCellVoltVld_flg/1 -> OCVCorrect/5(GbNDP_ReadMinCellVoltVld_flg)
  PackCurrCal/1(LcSOC_PackCurrAvg_A) -> LcSOC_PackCurrAvg_A/1
  GcRTC_SleepTime_min/1 -> Bus Creator/1  "GcRTC_SleepTime_min"
  GeMSM_BMUState_enum/1 -> Bus Creator/2  "GeMSM_BMUState_enum"
  GcCDP_MaxCellVolt_mV/1 -> Bus Creator/3  "GcCDP_MaxCellVolt_mV"
  GcCDP_MinCellVolt_mV/1 -> Bus Creator/4  "GcCDP_MinCellVolt_mV"
  GbNDP_ReadMaxCellSOCVld_flg/1 -> Bus Creator/5  "GbNDP_ReadMaxCellSOCVld_flg"
  GbNDP_ReadMinCellSOCVld_flg/1 -> Bus Creator/6  "GbNDP_ReadMinCellSOCVld_flg"
  GbCDP_SumCellVoltVld_flg/1 -> Bus Creator/7  "GbCDP_SumCellVoltVld_flg"
  GbUDS_MnlSOCCorrd_flg/1 -> Bus Creator/8  "GbUDS_MnlSOCCorrd_flg"
  Bus Selector5/1 -> OCVCorrect_On/1(GcRTC_SleepTime_min)  "<GcRTC_SleepTime_min>"
  Bus Selector5/2 -> OCVCorrect_On/2(GbNDP_ReadMaxCellSOCVld_flg)  "<GbNDP_ReadMaxCellSOCVld_flg>"
  Bus Selector5/3 -> OCVCorrect_On/3(GbNDP_ReadMinCellSOCVld_flg)  "<GbNDP_ReadMinCellSOCVld_flg>"
  Bus Selector5/4 -> OCVCorrect_On/4(GcCDP_MaxCellVolt_mV)  "<GcCDP_MaxCellVolt_mV>"
  Bus Selector5/5 -> OCVCorrect_On/5(GcCDP_MinCellVolt_mV)  "<GcCDP_MinCellVolt_mV>"
  Bus Selector5/6 -> OCVCorrect_On/6(GeMSM_BMUState_enum)  "<GeMSM_BMUState_enum>"
  Bus Selector5/7 -> OCVCorrect_On/7(GbCDP_SumCellVoltVld_flg)  "<GbCDP_SumCellVoltVld_flg>"
  Bus Selector5/8 -> OCVCorrect_On/8(GbUDS_MnlSOCCorrd_flg)  "<GbUDS_MnlSOCCorrd_flg>"
  GcHDP_PackCrnt_A/1 -> Bus Creator/9  "GcHDP_PackCrnt_A"
  Bus Selector3/1 -> PackCurrCal/1(GcHDP_PackCrnt_A)  "<GcHDP_PackCrnt_A>"
  GbHDP_PackCrntVld_flg/1 -> Bus Creator/10  "GbHDP_PackCrntVld_flg"
  Bus Selector4/1 -> SOCDepla_Correct/1(GcHDP_PackCrnt_A)  "<GcHDP_PackCrnt_A>"
  Bus Selector4/2 -> SOCDepla_Correct/2(GbHDP_PackCrntVld_flg)  "<GbHDP_PackCrntVld_flg>"
  Bus Selector4/3 -> SOCDepla_Correct/3(GcCDP_MaxCellVolt_mV)  "<GcCDP_MaxCellVolt_mV>"
  Bus Selector4/4 -> SOCDepla_Correct/4(GcCDP_MinCellVolt_mV)  "<GcCDP_MinCellVolt_mV>"
  Bus Selector4/5 -> SOCDepla_Correct/5(GbCDP_SumCellVoltVld_flg)  "<GbCDP_SumCellVoltVld_flg>"
  Bus Selector4/6 -> SOCDepla_Correct/6(GcRTC_SleepTime_min)  "<GcRTC_SleepTime_min>"
  SOCDepla_Correct/1(GcSOC_CellDeplaTi_min) -> GcSOC_CellDeplaTi_min/1
  SOCDepla_Correct/2(GbSOC_SOCDeplaTiReach_flg) -> GbSOC_SOCDeplaTiReach_flg/1
  Bus Selector6/1 -> ZeroSOC_flg/1(GcCDP_MinCellVolt_mV)  "<GcCDP_MinCellVolt_mV>"
  ZeroSOC_flg/1(LbSOC_ZeroSOCCorrect_flg) -> LbSOC_ZeroSOCCorrect_flg/1, EdgeRising3/1
  EdgeRising3/1 -> ZeroSOCCorrect/Enable
  EdgeRising4/1 -> DCStepChrgCorrect/Enable
  GbDCC_ChrgSt2StepChrg_flg/1 -> EdgeRising4/1  "GbDCC_ChrgSt2StepChrg_flg"
  GbACC_ChrgSt2StepChrg_flg/1 -> EdgeRising5/1  "GbACC_ChrgSt2StepChrg_flg"
  EdgeRising5/1 -> ACStepChrgCorrect/Enable
  GcCDP_MinCellTemp_C/1 -> Moving Average/1(u)  "GcCDP_MinCellTemp_C"
  Moving Average/1(y) -> LcCDP_MinCellAvgFitTemp_C/1, ZeroSOC_flg/3(LcCDP_MinCellAvgFitTemp_C), ACChrgFinishCorrect/1(LcCDP_MinCellAvgFitTemp_C), DCChrgFinishCorrect/1(LcCDP_MinCellAvgFitTemp_C)  "LcCDP_MinCellAvgFitTemp_C"
  Constant7/1 -> Moving Average/2(R)
  Bus Selector6/2 -> ZeroSOC_flg/2(GcHDP_PackCrnt_A)  "<GcHDP_PackCrnt_A>"
  GcADP_YearSet_Yr/1 -> Bus Creator/11  "GcADP_YearSet_Yr"
  GbISP_TF37FTiout_flg/1 -> Bus Creator/12  "GbISP_TF37FTiout_flg"
  Bus Selector5/9 -> OCVCorrect_On/9(GcADP_YearSet_Yr)  "<GcADP_YearSet_Yr>"
  Bus Selector5/10 -> OCVCorrect_On/10(GbISP_TF37FTiout_flg)  "<GbISP_TF37FTiout_flg>"
  GeUDS_CapSel_enum/1 -> Bus Creator/13  "GeUDS_CapSel_enum"
  Bus Selector4/7 -> SOCDepla_Correct/7(GeUDS_CapSel_enum)  "<GeUDS_CapSel_enum>"
  Bus Selector/3 -> OCVCorrect/3(GeUDS_CapSel_enum)  "<GeUDS_CapSel_enum>"

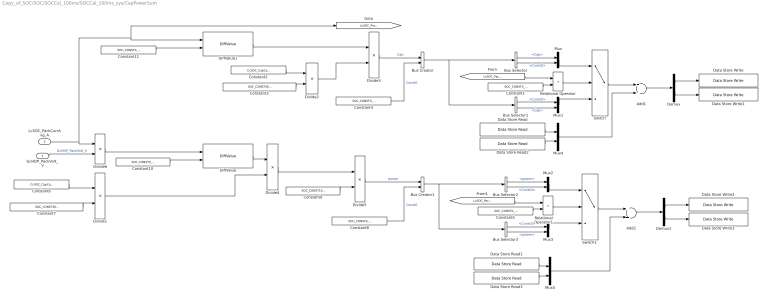
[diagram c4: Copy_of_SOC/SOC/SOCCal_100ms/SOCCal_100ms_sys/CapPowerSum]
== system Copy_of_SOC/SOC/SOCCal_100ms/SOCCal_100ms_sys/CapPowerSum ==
  GcHDP_PackVolt_V : Inport
  LcSOC_PackCurrAvg_A : Inport  Port=2
  Add1 : Sum  AccumDataTypeStr=single  OutDataTypeStr=single
  Add2 : Sum  AccumDataTypeStr=single  OutDataTypeStr=single
  Bus Creator : BusCreator  Inputs=2
  Bus Creator1 : BusCreator  Inputs=2
  Bus Selector : BusSelector  OutputSignals=Cap,Const0
  Bus Selector1 : BusSelector  OutputSignals=Const0,Cap
  Bus Selector2 : BusSelector  OutputSignals=power,Const0
  Bus Selector3 : BusSelector  OutputSignals=Const0,power
  Constant{1,4..5,8,10..11} (6 alike) : Constant  Value=SOC_CONST0_NUMB
  Constant2 : Constant  Value=CcSOC_CapCalcCycl_ms
  Constant3 : Constant  Value=SOC_CONST3600000_NUMB
  Constant6 : Constant  Value=CcSOC_CapCalcCycl_ms
  Constant7 : Constant  Value=SOC_CONST3600000_NUMB
  Constant9 : Constant  Value=SOC_CONST1000_NUMB
  Data Store Read : AIWAYS_Powertrain_BMS_lib/Signals/Data Store Read  Priority=0  DSR=EcNVM_TotalChrgCap_Ah
  Data Store Read1 : AIWAYS_Powertrain_BMS_lib/Signals/Data Store Read  Priority=0  DSR=EcNVM_TotalChrgPwr_kWh
  Data Store Read2 : AIWAYS_Powertrain_BMS_lib/Signals/Data Store Read  Priority=0  DSR=EcNVM_TotalDischrgCap_Ah
  Data Store Read3 : AIWAYS_Powertrain_BMS_lib/Signals/Data Store Read  Priority=0  DSR=EcNVM_TotalDischrgPwr_kWh
  Data Store Write : AIWAYS_Powertrain_BMS_lib/Signals/Data Store Write  DSW=EcNVM_TotalChrgCap_Ah
  Data Store Write1 : AIWAYS_Powertrain_BMS_lib/Signals/Data Store Write  DSW=EcNVM_TotalDischrgCap_Ah
  Data Store Write2 : AIWAYS_Powertrain_BMS_lib/Signals/Data Store Write  DSW=EcNVM_TotalChrgPwr_kWh
  Data Store Write3 : AIWAYS_Powertrain_BMS_lib/Signals/Data Store Write  DSW=EcNVM_TotalDischrgPwr_kWh
  Demux : Demux  Outputs=2
  Demux1 : Demux  Outputs=2
  DiffValue : AIWAYS_Powertrain_BMS_lib/Mathematical Functions/DiffValue
  DiffValue1 : AIWAYS_Powertrain_BMS_lib/Mathematical Functions/DiffValue
  Divide1 : Product  Inputs=*/  OutDataTypeStr=single
  Divide2 : Product  Inputs=*/  OutDataTypeStr=single
  Divide3 : Product  Inputs=**  OutDataTypeStr=single
  Divide4 : Product  Inputs=**  OutDataTypeStr=single
  Divide5 : Product  Inputs=*/  OutDataTypeStr=single
  Divide6 : Product  Inputs=**  OutDataTypeStr=single
  Mux{,1..5} (6 alike) : Mux  Inputs=2
  Relational Operator : RelationalOperator  Operator=<  OutDataTypeStr=boolean
  Relational Operator1 : RelationalOperator  Operator=<  OutDataTypeStr=boolean
  Switch : Switch  Criteria=u2 ~= 0
  Switch1 : Switch  Criteria=u2 ~= 0
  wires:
  Data Store Read3/1 -> Mux5/2
  Data Store Read1/1 -> Mux5/1
  Data Store Read2/1 -> Mux4/2
  Data Store Read/1 -> Mux4/1
  Add2/1 -> Demux1/1
  Mux4/1 -> Add1/2
  GcHDP_PackVolt_V/1 -> Divide6/2  "GcHDP_PackVolt_V"
  Demux/2 -> Data Store Write1/1
  Demux/1 -> Data Store Write/1
  Divide5/1 -> Bus Creator1/1  "power"
  Divide4/1 -> Divide5/1
  Bus Selector3/2 -> Mux3/2  "<power>"
  Constant9/1 -> Divide5/2
  Bus Selector1/1 -> Mux1/1  "<Const0>"
  Bus Selector3/1 -> Mux3/1  "<Const0>"
  Bus Selector1/2 -> Mux1/2  "<Cap>"
  Mux2/1 -> Switch1/1
  Relational Operator1/1 -> Switch1/2
  Constant7/1 -> Divide1/2
  Constant5/1 -> Relational Operator1/2
  Divide1/1 -> Divide4/2
  Bus Creator1/1 -> Bus Selector3/1, Bus Selector2/1
  Demux1/1 -> Data Store Write2/1
  Divide6/1 -> DiffValue/1
  Bus Selector2/2 -> Mux2/2  "<Const0>"
  Mux5/1 -> Add2/2
  Demux1/2 -> Data Store Write3/1
  Constant6/1 -> Divide1/1
  [LcSOC_PackCurrAvg_A] -> Relational Operator1/1
  Mux3/1 -> Switch1/3
  Bus Selector2/1 -> Mux2/1  "<power>"
  DiffValue/1 -> Divide4/1
  Constant8/1 -> Bus Creator1/2  "Const0"
  Switch1/1 -> Add2/1
  Add1/1 -> Demux/1
  Constant3/1 -> Divide2/2
  Divide2/1 -> Divide3/2
  LcSOC_PackCurrAvg_A/1 -> [LcSOC_PackCurrAvg_A], DiffValue1/1, Divide6/1
  Mux/1 -> Switch/1
  Bus Selector/2 -> Mux/2  "<Const0>"
  Divide3/1 -> Bus Creator/1  "Cap"
  [LcSOC_PackCurrAvg_A] -> Relational Operator/1
  Mux1/1 -> Switch/3
  DiffValue1/1 -> Divide3/1
  Constant4/1 -> Bus Creator/2  "Const0"
  Bus Selector/1 -> Mux/1  "<Cap>"
  Constant1/1 -> Relational Operator/2
  Relational Operator/1 -> Switch/2
  Constant2/1 -> Divide2/1
  Bus Creator/1 -> Bus Selector/1, Bus Selector1/1
  Switch/1 -> Add1/1
  Constant10/1 -> DiffValue/2
  Constant11/1 -> DiffValue1/2

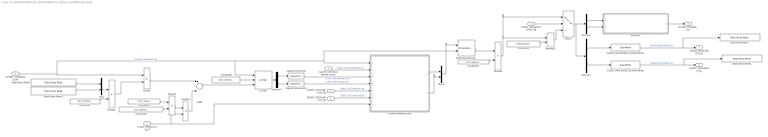
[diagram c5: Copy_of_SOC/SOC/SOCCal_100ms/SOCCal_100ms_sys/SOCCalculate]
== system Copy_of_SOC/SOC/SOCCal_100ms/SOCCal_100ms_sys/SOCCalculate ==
  LcSOC_PackCurrAvg_A : Inport
  LbSOC_ZeroSOCCorrect_flg : Inport  Port=2
  GeCTC_CtrCtlConnMode_enum : Inport  Port=3
  GcSOH_CurrBatCap_Ah : Inport  Port=4
  GbACC_ACChrgFinish_flg : Inport  Port=5
  GbDCC_DCChrgFinish_flg : Inport  Port=6
  Add1 : Sum  Inputs=+-  AccumDataTypeStr=single  OutDataTypeStr=single
  ChrgFinishBeforeLimit : Subsystem
  Constant1 : Constant  Value=SOC_CONST100_NUMB
  Constant2 : Constant  Value=CcSOC_CapCalcCycl_ms
  Constant3 : Constant  Value=SOC_CONST3600000_NUMB
  Constant4 : Constant  Value=CcSOC_ZeroMinSOC_pct
  Constant5 : Constant  Value=SOC_CONST100_NUMB
  Constant8 : Constant  Value=SOC_CONST0_NUMB
  Data Store Read : AIWAYS_Powertrain_BMS_lib/Signals/Data Store Read  Priority=0  DSR=EcNVM_MaxCellSOC_pct
  Data Store Read1 : AIWAYS_Powertrain_BMS_lib/Signals/Data Store Read  Priority=0  DSR=EcNVM_MinCellSOC_pct
  Data Store Write : AIWAYS_Powertrain_BMS_lib/Signals/Data Store Write  DSW=EcNVM_MaxCellSOC_pct
  Data Store Write1 : AIWAYS_Powertrain_BMS_lib/Signals/Data Store Write  DSW=EcNVM_MinCellSOC_pct
  Demux1 : Demux  Outputs=2
  Demux2 : Demux  Outputs=2
  Demux3 : Demux  Outputs=2
  Divide : Product  Inputs=**  OutDataTypeStr=single
  Divide1 : Product  Inputs=*/  OutDataTypeStr=single
  Divide2 : Product  Inputs=*/  OutDataTypeStr=single
  Divide3 : Product  Inputs=**  OutDataTypeStr=single
  Divide5 : Product  Inputs=**  OutDataTypeStr=Inherit: Inherit via back propagation
  GcSOC_MaxCellSOC_pctOverWrite : AIWAYS_Powertrain_BMS_lib/Signals/OverWrite  OverWrite_Value=CcSOC_MaxCellSOCOvr_pct  OverWrite_flag=CbSOC_MaxCellSOCOvrSwt_flg
  GcSOC_MinCellSOC_pctOverWrite : AIWAYS_Powertrain_BMS_lib/Signals/OverWrite  OverWrite_Value=CcSOC_MinCellSOCOvr_pct  OverWrite_flag=CbSOC_MinCellSOCOvrSwt_flg
  Limiter : AIWAYS_Powertrain_BMS_lib/Nonlinear Blocks/Limiter
  MinMax2 : MinMax  Function=max  Inputs=2  OutDataTypeStr=Inherit: Inherit via back propagation  RndMeth=Zero
  Mux : Mux  Inputs=2
  Mux2 : Mux  Inputs=2
  PackSOC : Subsystem
  Protected Division : AIWAYS_Powertrain_BMS_lib/Arithmetic Operators/Protected Division
  Signal Conversion : SignalConversion  ConversionOutput=Contiguous copy  OverrideOpt=off
  Signal Conversion1 : SignalConversion  ConversionOutput=Contiguous copy  OverrideOpt=off
  Switch : Switch  Criteria=u2 ~= 0  Threshold=1  RndMeth=Zero
  GcSOC_MaxCellSOC_pct : Outport
  GcSOC_MinCellSOC_pct : Outport  Port=2
  GcSOC_PackSOC_pct : Outport  Port=3
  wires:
  GcSOC_MinCellSOC_pctOverWrite/1 -> GcSOC_MinCellSOC_pct/1, Data Store Write1/1  "GcSOC_MinCellSOC_pct"
  GcSOC_MaxCellSOC_pctOverWrite/1 -> GcSOC_MaxCellSOC_pct/1, Data Store Write/1  "GcSOC_MaxCellSOC_pct"
  Add1/1 -> Limiter/3
  Limiter/1 -> Demux3/1
  Constant2/1 -> Divide2/1
  Constant3/1 -> Divide2/2
  GcSOH_CurrBatCap_Ah/1 -> Protected Division/2, ChrgFinishBeforeLimit/1(GcSOH_CurrBatCap_Ah), Limiter/1, Divide/1  "GcSOH_CurrBatCap_Ah"
  Protected Division/1 -> Divide5/1
  Constant5/1 -> Divide5/2
  Demux2/1 -> PackSOC/1(GcSOC_MaxCellSOC_pct)
  Demux2/2 -> PackSOC/2(GcSOC_MinCellSOC_pct)
  PackSOC/1(GcSOC_PackSOC_pct) -> GcSOC_PackSOC_pct/1
  Mux2/1 -> Protected Division/1
  Demux3/1 -> Signal Conversion/1
  Demux3/2 -> Signal Conversion1/1
  GeCTC_CtrCtlConnMode_enum/1 -> ChrgFinishBeforeLimit/2(GeCTC_CtrCtlConnMode_enum)  "GeCTC_CtrCtlConnMode_enum"
  ChrgFinishBeforeLimit/1(LcSOC_MaxCellCap_Ah) -> Mux2/1
  ChrgFinishBeforeLimit/2(LcSOC_MinCellCap_Ah) -> Mux2/2
  Demux1/1 -> GcSOC_MaxCellSOC_pctOverWrite/1
  Demux1/2 -> GcSOC_MinCellSOC_pctOverWrite/1
  GbACC_ACChrgFinish_flg/1 -> ChrgFinishBeforeLimit/5(GbACC_ACChrgFinish_flg)  "GbACC_ACChrgFinish_flg"
  Constant1/1 -> Divide1/2
  Divide1/1 -> Divide/2
  Mux/1 -> Divide1/1
  Data Store Read/1 -> Mux/1
  Data Store Read1/1 -> Mux/2
  GbDCC_DCChrgFinish_flg/1 -> ChrgFinishBeforeLimit/6(GbDCC_DCChrgFinish_flg)  "GbDCC_DCChrgFinish_flg"
  Divide2/1 -> Divide3/1
  LcSOC_PackCurrAvg_A/1 -> ChrgFinishBeforeLimit/7(LcSOC_PackCurrAvg_A), Divide3/2
  Divide/1 -> Add1/1
  Divide3/1 -> Add1/2
  Constant8/1 -> Limiter/2
  Signal Conversion/1 -> ChrgFinishBeforeLimit/3(LcSOC_MaxCellCapIn_Ah)  "LcSOC_MaxCellCapIn_Ah"
  Signal Conversion1/1 -> ChrgFinishBeforeLimit/4(LcSOC_MinCellCapIn_Ah)  "LcSOC_MinCellCapIn_Ah"
  LbSOC_ZeroSOCCorrect_flg/1 -> Switch/2
  Switch/1 -> Demux1/1, Demux2/1
  Divide5/1 -> MinMax2/1, Switch/1
  MinMax2/1 -> Switch/3
  Constant4/1 -> MinMax2/2

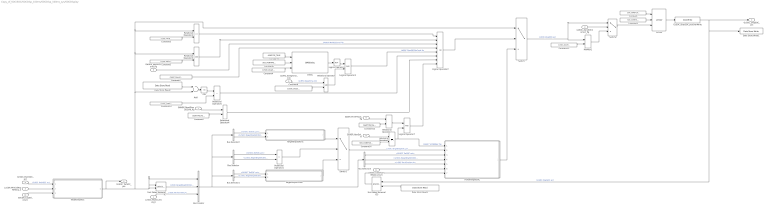
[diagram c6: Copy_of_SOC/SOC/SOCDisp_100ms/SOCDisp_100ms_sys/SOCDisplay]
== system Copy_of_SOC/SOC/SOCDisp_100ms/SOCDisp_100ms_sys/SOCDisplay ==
  LcSOC_PackCurrAvg_A : Inport
  LbSOC_ZeroSOCCorrect_flg : Inport  Port=2
  LcCDP_MinCellAvgFitTemp_C : Inport  Port=3
  GcSOC_PackSOC_pct : Inport  Port=4
  GcRTC_SleepTime_min : Inport  Port=5
  GbUDS_MnlSOCCorrd_flg : Inport  Port=6
  GbNDP_ReadDispSOCVld_flg : Inport  Port=7
  GcADP_YearSet_Yr : Inport  Port=8
  GbISP_TF37FTiout_flg : Inport  Port=9
  GeUDS_CapSel_enum : Inport  Port=10
  GeCTC_CtrCtlConnMode_enum : Inport  Port=11
  Abs : Abs
  Add : Sum  Inputs=+-  OutDataTypeStr=single
  Bus Creator : BusCreator  Inputs=3
  Bus Selector : BusSelector  OutputSignals=GcSOC_TarSOC_pct,LcSOC_TargetDispSOCOld_pct
  Bus Selector1 : BusSelector  OutputSignals=GcSOC_TarSOC_pct,LcSOC_TargetDispSOCOld_pct
  Bus Selector2 : BusSelector  OutputSignals=GcSOC_TarSOC_pct,LcSOC_TargetDispSOCOld_pct
  Bus Selector3 : BusSelector  OutputSignals=GcSOC_TarSOC_pct,LcSOC_TargetDispSOCOld_pct,LcSOC_PackCurrAvg_A
  Constant : Constant  Value=SOC_CONST100_NUMB
  Constant1 : Constant  Value=CbSOC_ManuOCVCorrect_flg
  Constant10 : Constant  Value=CcSOC_DispSOCErr_pct
  Constant11 : Constant  Value=CcSOC_ZeroMinSOC_pct
  Constant12 : Constant  Value=ASWTYPE_FALSE
  Constant14 : Constant  Value=SOC_CONST2080_NUMB
  Constant2 : Constant  Value=SOC_CONST0_NUMB
  Constant3 : Constant  Value=CcSOC_MinFlwDispSOC_pct
  Constant4 : Constant  Value=CcSOC_DispSOCCordRunTi_ms
  Constant5 : Constant  Value=CcSOC_MaxFlwDispSOC_pct
  Constant6 : Constant  Value=SOC_RUNTIME100_MS
  Constant7 : Constant  Value=ASWTYPE_TRUE
  Constant8 : Constant  Value=CcSOC_DispSOCChgSleepTime_min
  Constant9 : Constant  Value=ASWTYPE_FALSE
  Data Store Read1 : AIWAYS_Powertrain_BMS_lib/Signals/Data Store Read  Priority=0  DSR=EcNVM_DispSOC_pct
  Data Store Read2 : AIWAYS_Powertrain_BMS_lib/Signals/Data Store Read  Priority=0  DSR=EcNVM_DispSOC_pct
  Data Store Write1 : AIWAYS_Powertrain_BMS_lib/Signals/Data Store Write  DSW=EcNVM_DispSOC_pct
  Delay : AIWAYS_Powertrain_BMS_lib/Debounce & Delay/BMSDelay
  FollowTargetSOC : Subsystem
  GcSOC_DispSOC_pctOverWrite : AIWAYS_Powertrain_BMS_lib/Signals/OverWrite  OverWrite_Value=CcSOC_DispSOCOvr_pct  OverWrite_flag=CbSOC_DispSOCOvrSwt_flg
  Limiter : AIWAYS_Powertrain_BMS_lib/Nonlinear Blocks/Limiter
  Logical Operator1 : Logic  Operator=NOT  AllPortsSameDT=off  OutDataTypeStr=boolean
  Logical Operator2 : Logic  Operator=OR  Inputs=8  AllPortsSameDT=off  OutDataTypeStr=boolean
  Logical Operator3 : Logic  AllPortsSameDT=off  OutDataTypeStr=boolean
  Logical Operator7 : Logic  AllPortsSameDT=off  OutDataTypeStr=boolean
  MinMax1 : MinMax  Function=max  Inputs=2  OutDataTypeStr=Inherit: Inherit via back propagation  RndMeth=Zero
  Relational Operator : RelationalOperator  OutDataTypeStr=boolean
  Relational Operator1 : RelationalOperator  Operator=>  OutDataTypeStr=boolean
  Relational Operator2 : RelationalOperator  Operator=<=  OutDataTypeStr=boolean
  Relational Operator3 : RelationalOperator  OutDataTypeStr=boolean
  Relational Operator4 : RelationalOperator  Operator===  OutDataTypeStr=boolean
  Relational Operator5 : RelationalOperator  Operator=>  OutDataTypeStr=boolean
  Relational Operator7 : RelationalOperator  Operator===  OutDataTypeStr=boolean
  Relational Operator8 : RelationalOperator  Operator===  OutDataTypeStr=boolean
  Switch : Switch  Criteria=u2 ~= 0  Threshold=1  RndMeth=Zero
  Switch1 : Switch  Criteria=u2 ~= 0  Threshold=1  RndMeth=Zero
  Switch2 : Switch  Criteria=u2 ~= 0  Threshold=1  RndMeth=Zero
  TargetDispSOC : Subsystem
  TargetDispSOCDec : Subsystem
  TargetDispSOCInc : Subsystem
  Unit Delay External IC : AIWAYS_Powertrain_BMS_lib/Delay Blocks/Unit Delay External IC
  Unit Delay External IC3 : AIWAYS_Powertrain_BMS_lib/Delay Blocks/Unit Delay External IC
  GcSOC_TarSOC_pct : Outport
  GcSOC_DispSOC_pct : Outport  Port=2
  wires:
  GcSOC_PackSOC_pct/1 -> TargetDispSOC/1(GcSOC_PackSOC_pct)  "GcSOC_PackSOC_pct"
  GbUDS_MnlSOCCorrd_flg/1 -> Logical Operator2/3  "GbUDS_MnlSOCCorrd_flg"
  Constant7/1 -> Delay/1
  Constant6/1 -> Delay/2
  Constant4/1 -> Delay/3
  GcRTC_SleepTime_min/1 -> Relational Operator/1  "GcRTC_SleepTime_min"
  Relational Operator/1 -> Logical Operator3/2
  Data Store Read1/1 -> Unit Delay External IC3/2
  Constant5/1 -> Relational Operator3/2
  Constant8/1 -> Relational Operator/2
  Relational Operator2/1 -> Logical Operator2/1
  Constant3/1 -> Relational Operator2/2
  Relational Operator3/1 -> Logical Operator2/2
  TargetDispSOCInc/1(LcSOC_TargetDispSOCInc_pct) -> Switch1/1
  Bus Selector3/2 -> FollowTargetSOC/4(LcSOC_TargetDispSOCOld_pct)  "<LcSOC_TargetDispSOCOld_pct>"
  Bus Selector/1 -> Relational Operator1/1  "<GcSOC_TarSOC_pct>"
  Bus Selector1/2 -> TargetDispSOCDec/2(LcSOC_TargetDispSOCOld_pct)  "<LcSOC_TargetDispSOCOld_pct>"
  Bus Creator/1 -> Bus Selector3/1, Bus Selector1/1, Bus Selector2/1, Bus Selector/1
  Bus Selector/2 -> Relational Operator1/2  "<LcSOC_TargetDispSOCOld_pct>"
  Bus Selector2/2 -> TargetDispSOCInc/2(LcSOC_TargetDispSOCOld_pct)  "<LcSOC_TargetDispSOCOld_pct>"
  Bus Selector3/3 -> FollowTargetSOC/5(LcSOC_PackCurrAvg_A)  "<LcSOC_PackCurrAvg_A>"
  Bus Selector2/1 -> TargetDispSOCInc/1(GcSOC_TarSOC_pct)  "<GcSOC_TarSOC_pct>"
  Switch1/1 -> FollowTargetSOC/2(LcSOC_TargetDispSOC_pct)  "LcSOC_TargetDispSOC_pct"
  Unit Delay External IC3/1 -> FollowTargetSOC/7(LcSOC_OldDispSOC_pct)
  FollowTargetSOC/1(LcSOC_FilterTarDispSOC_pct) -> Switch/3
  Bus Selector3/1 -> FollowTargetSOC/3(GcSOC_TarSOC_pct)  "<GcSOC_TarSOC_pct>"
  Relational Operator1/1 -> Switch1/2
  Delay/1 -> Logical Operator1/1
  LcSOC_PackCurrAvg_A/1 -> Bus Creator/3  "LcSOC_PackCurrAvg_A"
  Bus Selector1/1 -> TargetDispSOCDec/1(GcSOC_TarSOC_pct)  "<GcSOC_TarSOC_pct>"
  Unit Delay External IC/1 -> Bus Creator/2  "LcSOC_TargetDispSOCOld_pct"
  GcSOC_DispSOC_pctOverWrite/1 -> Data Store Write1/1, Unit Delay External IC3/1, GcSOC_DispSOC_pct/1  "GcSOC_DispSOC_pct"
  Logical Operator2/1 -> Switch/2
  Logical Operator1/1 -> Logical Operator3/1
  TargetDispSOCDec/1(LcSOC_TargetDispSOCDec_pct) -> Switch1/3
  Logical Operator3/1 -> Logical Operator2/5  "LbSOC_DispSOCSlpCond_flg"
  Constant1/1 -> Logical Operator2/4
  Constant/1 -> Limiter/1
  Constant2/1 -> Limiter/2
  Constant9/1 -> Relational Operator4/2
  GbNDP_ReadDispSOCVld_flg/1 -> Relational Operator4/1
  Data Store Read2/1 -> Add/1
  Add/1 -> Abs/1
  Constant10/1 -> Relational Operator5/2
  Abs/1 -> Relational Operator5/1
  TargetDispSOC/1(GcSOC_TarSOC_pct) -> Add/2, Relational Operator3/1, Relational Operator2/1, Switch/1, Bus Creator/1, Unit Delay External IC/1, Unit Delay External IC/2, GcSOC_TarSOC_pct/1
  Relational Operator4/1 -> Logical Operator2/7
  Relational Operator5/1 -> Logical Operator2/6
  LcCDP_MinCellAvgFitTemp_C/1 -> TargetDispSOC/2(LcCDP_MinCellAvgFitTemp_C)
  LbSOC_ZeroSOCCorrect_flg/1 -> Switch2/2
  Switch/1 -> Switch2/1, MinMax1/1  "LcSOC_DispSOC_pct"
  Switch2/1 -> Limiter/3
  Limiter/1 -> GcSOC_DispSOC_pctOverWrite/1
  MinMax1/1 -> Switch2/3
  Constant11/1 -> MinMax1/2
  Constant14/1 -> Relational Operator8/2
  GcADP_YearSet_Yr/1 -> Relational Operator8/1
  GbISP_TF37FTiout_flg/1 -> Relational Operator7/1
  Constant12/1 -> Relational Operator7/2
  Logical Operator7/1 -> Logical Operator2/8
  GeUDS_CapSel_enum/1 -> TargetDispSOC/3(GeUDS_CapSel_enum)
  GeCTC_CtrCtlConnMode_enum/1 -> FollowTargetSOC/6(GeCTC_CtrCtlConnMode_enum)
  Relational Operator8/1 -> FollowTargetSOC/1(LbSOC_Yr2080Rec_flg), Logical Operator7/2  "LbSOC_Yr2080Rec_flg"
  Relational Operator7/1 -> Logical Operator7/1

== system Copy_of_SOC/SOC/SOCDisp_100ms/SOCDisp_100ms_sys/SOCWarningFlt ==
  GcSOC_DispSOC_pct : Inport
  HighAlarm : Subsystem
  HighWarning : Subsystem
  LowAlarm : Subsystem
  LowWarning : Subsystem
  GbSOC_SOCLowWarn_flg : Outport
  GbSOC_SOCHghWarn_flg : Outport  Port=2
  GbSOC_SOCHghAlrm_flg : Outport  Port=3
  GbSOC_SOCLowAlrm_flg : Outport  Port=4
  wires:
  GcSOC_DispSOC_pct/1 -> LowWarning/1(GcSOC_DispSOC_pct), HighWarning/1(GcSOC_DispSOC_pct), HighAlarm/1(GcSOC_DispSOC_pct), LowAlarm/1(GcSOC_DispSOC_pct)
  LowAlarm/1(GbSOC_SOCLowAlrm_flg) -> GbSOC_SOCLowAlrm_flg/1
  LowWarning/1(GbSOC_SOCLowWarn_flg) -> GbSOC_SOCLowWarn_flg/1
  HighAlarm/1(GbSOC_SOCHghAlrm_flg) -> GbSOC_SOCHghAlrm_flg/1
  HighWarning/1(GbSOC_SOCHghWarn_flg) -> GbSOC_SOCHghWarn_flg/1
